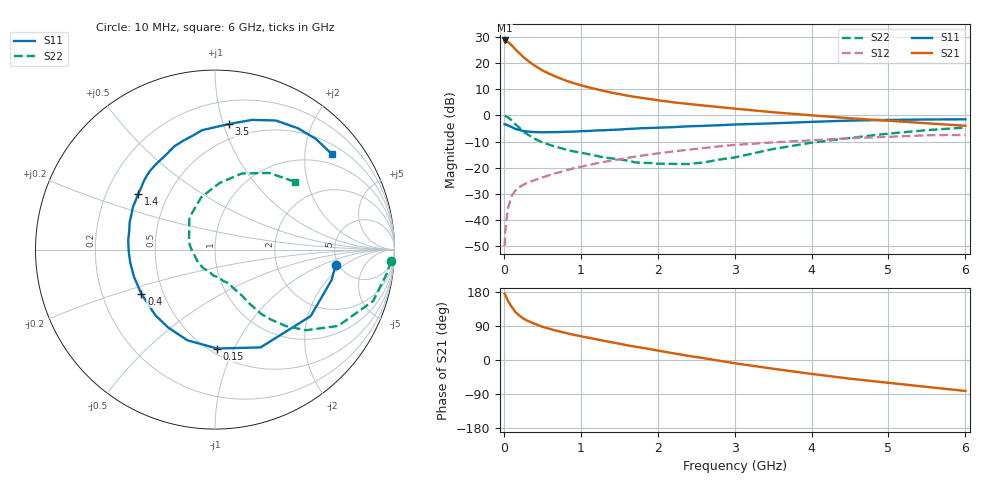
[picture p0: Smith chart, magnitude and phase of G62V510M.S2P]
! SIEMENS Small Signal Semiconductors
! BFG193
! Si NPN RF Bipolar Junction Transistor in SOT223
! VCE = 2.5 V  IC = 10 mA
! Common Emitter S-Parameters:  August  1996
# GHz  S  MA  R  50
!  f  S11  S21  S12  S22
! GHz  MAG  ANG  MAG  ANG  MAG  ANG  MAG  ANG
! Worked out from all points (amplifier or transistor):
!   36 points, 10 MHz to 6 GHz, reference 50 ohm
!   highest |S21| = 28.6 dB at 10 MHz (marker M1)
!   |S21| within 3 dB of that: start of sweep to 138 MHz
!   unconditionally stable (mu >= 1): 871.6 MHz to 2.616 GHz
!   at 250 MHz: K = 0.54, MSG = 24.4 dB, |S12| = -26.5 dB
!   at 1.4 GHz: K = 1.07, MAG = 11.4 dB, |S12| = -17.3 dB
!   at 6 GHz: K = 0.90, MSG = 1.7 dB, |S12| = -7.5 dB
!   S11 on the Smith chart (normalised r, x): 10 MHz: 4.70, -1.49; 150 MHz: 0.54, -0.86; 400 MHz: 0.38, -0.24; 1.4 GHz: 0.34, +0.29; 3.5 GHz: 0.38, +1.05; 6 GHz: 0.72, +2.63
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0.01  0.6769 -7.3  26.84 175.1  0.0032 90.9  0.981 -3.7
0.02  0.6717 -14.5  26.62 171.4  0.0065 85.1  0.9695 -7.5
0.05  0.6493 -34.8  25.34 157.4  0.0161 74.4  0.9265 -18.0
0.1  0.6013 -65.0  21.9 140.9  0.0287 64.9  0.8072 -31.8
0.15  0.5512 -88.8  18.16 126.7  0.0369 55.9  0.6781 -41.5
0.2  0.5282 -106.9  15.41 117.5  0.0425 52.6  0.5806 -47.2
0.25  0.5066 -120.9  13.09 109.9  0.0473 50.2  0.4982 -51.4
0.3  0.4942 -132.3  11.35 104.2  0.0515 49.3  0.4433 -54.2
0.4  0.4786 -148.9  8.892 95.5  0.0582 48.9  0.3587 -57.4
0.5  0.4763 -161.6  7.225 87.8  0.0654 48.9  0.3055 -59.3
0.6  0.4778 -171.1  6.123 81.9  0.0732 49.6  0.2729 -61.2
0.7  0.4808 -178.7  5.296 76.5  0.0806 49.7  0.2468 -63.6
0.9  0.4892 167.7  4.156 66.9  0.0971 49.1  0.2064 -67.3
1.1  0.5047 157.4  3.43 58.7  0.1125 48.2  0.1824 -74.8
1.4  0.5292 144.0  2.709 46.8  0.1369 44.8  0.1511 -86.8
1.7  0.5591 133.1  2.255 35.4  0.1626 40.9  0.1275 -102.7
2.2  0.5956 117.0  1.776 17.9  0.2052 31.7  0.1187 -141.1
2.8  0.6483 100.7  1.438 -1.9  0.2566 19.7  0.1433 169.8
3.5  0.7042 83.6  1.147 -23.0  0.3056 3.5  0.2281 128.8
4.5  0.795 64.8  0.88 -49.3  0.3678 -16.3  0.3715 86.1
5.5  0.8343 47.7  0.706 -71.0  0.4177 -40.1  0.5226 54.8
6  0.8409 39.3  0.633 -81.7  0.4232 -53.9  0.5858 40.1
